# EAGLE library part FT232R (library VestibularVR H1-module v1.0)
UART/FIFO IC
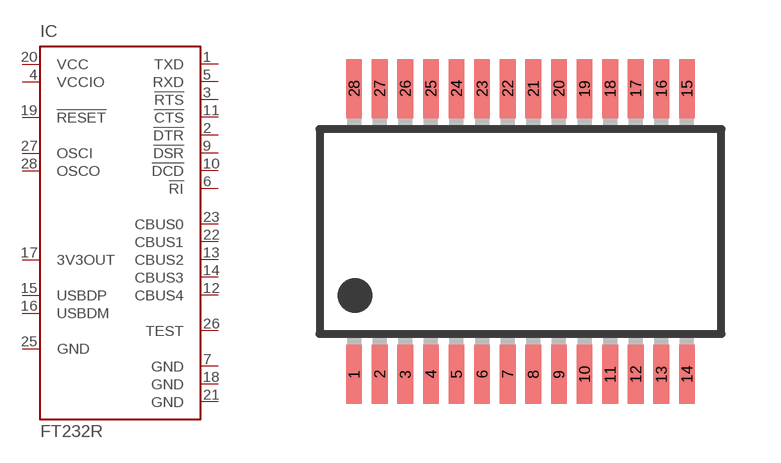
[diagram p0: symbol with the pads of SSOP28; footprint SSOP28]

Designator prefix IC

## FT232RL  [SSOP28]
1  TXD  out
2  !DTR  out
3  !RTS  out
4  VCCIO  pwr
5  RXD  in
6  !RI  in
7  GND  pwr
9  !DSR  in
10  !DCD  in
11  !CTS  in
12  CBUS4
13  CBUS2
14  CBUS3
15  USBDP
16  USBDM
17  3V3OUT  out
18  GND  pwr
19  !RESET  in
20  VCC  pwr
21  GND  pwr
22  CBUS1
23  CBUS0
25  GND  pwr
26  TEST  in
27  OSCI  in
28  OSCO  out

## Footprint SSOP28 (pad centres in mm)
Shrink Small Outline Package SSOP-28 http://www.ftdichip.com/Documents/DataSheets/DS_FT232R_v104.pdf
smd 0.4 x 1.5: 1 -4.225,-3.625; 2 -3.575,-3.625; 3 -2.925,-3.625; 4 -2.275,-3.625; 5 -1.625,-3.625; 6 -0.975,-3.625; 7 -0.325,-3.625; 8 0.325,-3.625; 9 0.975,-3.625; 10 1.625,-3.625; 11 2.275,-3.625; 12 2.925,-3.625; 13 3.575,-3.625; 14 4.225,-3.625; 15 4.225,3.625; 16 3.575,3.625; 17 2.925,3.625; 18 2.275,3.625; 19 1.625,3.625; 20 0.975,3.625; 21 0.325,3.625; 22 -0.325,3.625; 23 -0.975,3.625; 24 -1.625,3.625; 25 -2.275,3.625; 26 -2.925,3.625; 27 -3.575,3.625; 28 -4.225,3.625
